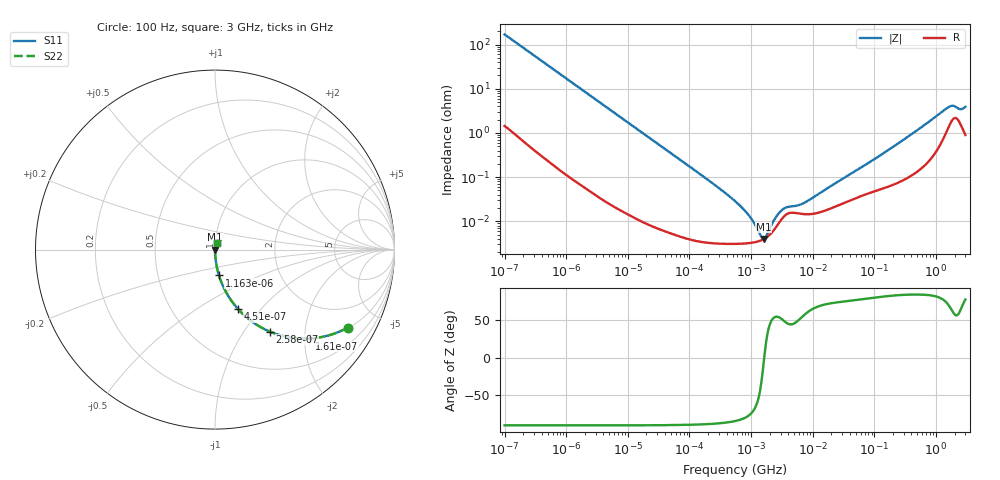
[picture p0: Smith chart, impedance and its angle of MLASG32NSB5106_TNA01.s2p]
! MLASG32NSB5106_TNA01  S-PARAMETER MODEL  ( Standard Model )
! Model Generated by TAIYO YUDEN Corporation (http://www.ty-top.com)
! Version 1.0
! TAIYO YUDEN Control No. 220601
! Copyright(c) 2009 TAIYO YUDEN CO.,LTD. All Rights Reserved.
! Product Description (link to TY-COMPAS)
! https://ds.yuden.co.jp/TYCOMPAS/or/detail?pn=MLASG32NSB5106KTNA01&u=M
! Products Name : Multilayer Ceramic Capacitors
! Characteristics :
!  Capacitance : 10 [uF] , Rated Voltage : 35 [V] , TCC : X5R
!  Case Size : 3.2 x 2.5 / 0.126 x 0.098 [mm/inch] , Thickness : 1.9 / 0.075 [mm/inch]
!  (Conditions: Temperature = 25 [degC] , DC Bias Voltage = 0 [V])
! External Node Assignments :
!  1  o---| |---o  2
! GND o---------o GND
! Frequency Range : 100Hz  -  3GHz  [ 401 STEP ]
# MHZ S RI R 50
! Freq[MHz].  S11 Real  S11 Imag  S21 Real  S21 Imag  S12 Real  S12 Imag  S22 Real  S22 Imag
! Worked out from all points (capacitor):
!   401 points, 100 Hz to 3 GHz, reference 50 ohm
!   read as one part in series: C = 9.37 uF near 109 Hz
!   lowest |Z| = 3.97 mohm at 1.607 MHz (marker M1)
!   series resonance near 1.632 MHz, so ESL is about 1 nH
!   S11 on the Smith chart (normalised r, x): 100 Hz: 1.03, -3.39; 161 Hz: 1.02, -2.12; 258 Hz: 1.01, -1.32; 451 Hz: 1.01, -0.76; 1.163 kHz: 1.00, -0.30; 3 GHz: 1.02, +0.08
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0.0001  0.7403 -0.4343  0.2597 0.4343  0.2597 0.4343  0.7403 -0.4343
0.000161  0.5287 -0.4952  0.4713 0.4952  0.4713 0.4952  0.5287 -0.4952
0.000258  0.3057 -0.457  0.6943 0.457  0.6943 0.457  0.3057 -0.457
0.000451  0.1273 -0.3298  0.8727 0.3298  0.8727 0.3298  0.1273 -0.3298
0.000664  0.0636 -0.2408  0.9364 0.2408  0.9364 0.2408  0.0636 -0.2408
0.001163  0.0222 -0.1441  0.9778 0.1441  0.9778 0.1441  0.0222 -0.1441
0.001788  0.00977 -0.0951  0.9902 0.0951  0.9902 0.0951  0.00977 -0.0951
0.005476  0.00122 -0.0315  0.9988 0.0315  0.9988 0.0315  0.00122 -0.0315
0.031977  9.62e-05 -0.00544  0.9999 0.00544  0.9999 0.00544  9.62e-05 -0.00544
0.231582  3.25e-05 -0.000742  1 0.000742  1 0.000742  3.25e-05 -0.000742
0.547723  3.09e-05 -0.000286  1 0.000286  1 0.000286  3.09e-05 -0.000286
1.09055  3.32e-05 -9.13e-05  1 9.13e-05  1 9.13e-05  3.32e-05 -9.13e-05
1.6065  3.96e-05 -3.53e-06  1 3.53e-06  1 3.53e-06  3.96e-05 -3.53e-06
2.171352  5.58e-05 6.6e-05  0.9999 -6.6e-05  0.9999 -6.6e-05  5.58e-05 6.6e-05
3.486191  0.000133 0.000147  0.9999 -0.000147  0.9999 -0.000147  0.000133 0.000147
6.368694  0.000148 0.00019  0.9999 -0.00019  0.9999 -0.00019  0.000148 0.00019
9.794414  0.000147 0.000301  0.9999 -0.000301  0.9999 -0.000301  0.000147 0.000301
175.1444  0.00064 0.00421  0.9994 -0.00421  0.9994 -0.00421  0.00064 0.00421
1573.002  0.0139 0.0349  0.9861 -0.0349  0.9861 -0.0349  0.0139 0.0349
1868.531  0.021 0.0345  0.979 -0.0345  0.979 -0.0345  0.021 0.0345
2525.516  0.0159 0.03  0.9841 -0.03  0.9841 -0.03  0.0159 0.03
3000  0.0103 0.0374  0.9897 -0.0374  0.9897 -0.0374  0.0103 0.0374
